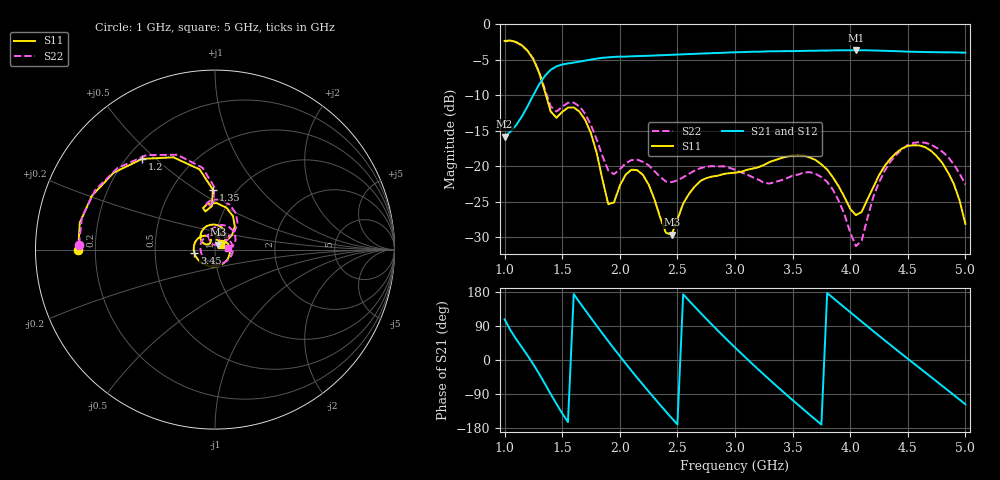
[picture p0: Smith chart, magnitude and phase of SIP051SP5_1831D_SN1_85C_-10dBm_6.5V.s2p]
# GHz  S  dB  R  50
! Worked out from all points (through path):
!   81 points, 1 GHz to 5 GHz, reference 50 ohm
!   highest |S21| = -3.67 dB at 4.05 GHz (marker M1); lowest = -15.8 dB at 1 GHz (marker M2)
!   lowest |S11| = -29.6 dB at 2.45 GHz (marker M3), VSWR 1.07, Z = 51.8 + j2.82 ohm
!   |S11| at or under -10 dB: 1.359 GHz to end of sweep
!   |S22| runs from -31.3 to -2.3 dB; largest |S21 - S12| = 0.0031
!   S11 on the Smith chart (normalised r, x): 1 GHz: 0.13, -0.00; 1.2 GHz: 0.26, +0.45; 1.35 GHz: 0.78, +0.59; 3.45 GHz: 0.79, -0.03; 5 GHz: 1.06, +0.05
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1  -2.36 -179.9  -15.83 107.3  -15.80 107.4  -2.40 177.9
1.2  -3.76 128.8  -11.55 11.5  -11.53 11.5  -3.74 125.9
1.35  -9.51 92.1  -7.27 -62.9  -7.25 -63.0  -9.18 90.5
1.45  -13.19 104.1  -5.94 -115.9  -5.92 -116.0  -12.31 99.4
1.55  -11.75 99.3  -5.53 -164.0  -5.52 -164.0  -11.07 93.8
1.7  -13.51 61.6  -5.13 131.4  -5.13 131.4  -12.64 60.1
1.9  -25.37 54.6  -4.67 49.6  -4.65 49.6  -20.61 50.1
2  -22.75 85.4  -4.57 10.2  -4.56 10.2  -20.45 66.2
2.2  -21.21 47.5  -4.47 -64.8  -4.47 -64.9  -19.40 48.4
2.35  -27.21 28.6  -4.38 -118.5  -4.36 -118.5  -21.50 38.9
2.45  -29.65 55.5  -4.31 -153.1  -4.30 -153.1  -22.26 40.4
2.6  -23.91 51.7  -4.21 156.8  -4.19 156.7  -21.10 37.9
2.75  -21.69 12.3  -4.12 108.8  -4.10 108.8  -20.10 19.6
3  -20.92 -63.2  -3.96 33.0  -3.95 32.8  -20.50 -31.2
3.2  -20.18 -116.4  -3.88 -24.3  -3.87 -24.3  -21.88 -91.4
3.45  -18.67 -170.8  -3.80 -92.5  -3.78 -92.6  -21.71 174.4
3.7  -19.13 140.8  -3.74 -157.7  -3.73 -157.8  -21.10 102.5
4.05  -26.91 128.7  -3.67 113.7  -3.67 113.6  -31.28 87.1
4.35  -18.94 135.8  -3.77 39.6  -3.78 39.5  -19.35 103.4
4.6  -17.08 91.7  -3.90 -20.6  -3.91 -20.7  -16.61 58.6
4.8  -19.56 55.6  -3.96 -68.6  -3.96 -68.5  -17.96 25.0
5  -28.15 37.1  -4.01 -116.8  -4.00 -116.9  -22.59 5.1
